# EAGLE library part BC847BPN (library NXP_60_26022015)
NPN/PNP general-purpose transistor pair in a very small SOT363 (SC-88) Surface-Mounted Device (SMD) plastic package. AAL Eindhoven MK
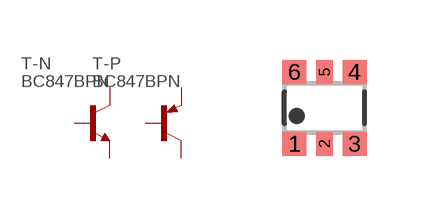
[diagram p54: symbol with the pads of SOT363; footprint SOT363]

Designator prefix T; gates -N=NPN -P=PNP

## BC847BPN  [SOT363]
1  -N:E  pas
2  -N:B  pas
3  -P:C  pas
4  -P:E  pas
5  -P:B  pas
6  -N:C  pas

## Footprint SOT363 (pad centres in mm)
SOT363 Plastic surface-mounted package; 6 leads JEDEC: -- IEC: -- JEITA: SC-88
smd 0.6 x 0.6: 1 -0.75,-0.9; 3 0.75,-0.9; 4 0.75,0.9; 6 -0.75,0.9
smd 0.4 x 0.6: 2 0,-0.9; 5 0,0.9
